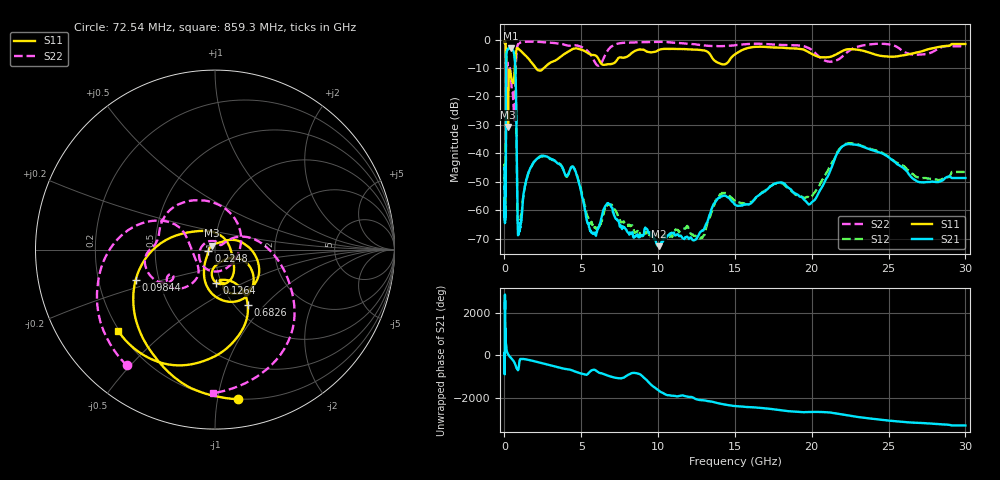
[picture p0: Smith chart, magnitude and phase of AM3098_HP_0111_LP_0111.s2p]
! Date/Time: Thu, Feb 28, 2019 8:38 AM
! Network Analyzer: Agilent Technologies E8364B Rev: A.07.50.67
! Sweep from 0.010 to 30.000 GHz, 1601 Points, Sweep Type: LOG
! Power Supply: 5.023 V, 0.001 A
# Hz S DB R 50
!freq MagS11 AngS11 MagS21 AngS21 MagS12 AngS12 MagS22 AngS22
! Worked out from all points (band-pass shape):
!   1601 points, 10 MHz to 30 GHz, reference 50 ohm
!   highest |S21| = -3.11 dB at 418 MHz (marker M1); lowest = -72.6 dB at 10.03 GHz (marker M2)
!   |S21| within 3 dB of the highest: 121.3 MHz to 660.5 MHz (539.2 MHz wide, 138 % of centre)
!   lowest |S11| = -30.7 dB at 231.6 MHz (marker M3), VSWR 1.06, Z = 48.1 + j2.15 ohm
!   |S11| at or under -10 dB: 102.2 MHz to 671.5 MHz (569.3 MHz wide, 147 % of centre); 2.04 GHz to 2.554 GHz (513.5 MHz wide, 22.4 % of centre)
!   |S22| runs from -28.3 to -0.6 dB; largest |S21 - S12| = 0.011
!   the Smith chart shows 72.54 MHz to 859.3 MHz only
!   S11 on the Smith chart (normalised r, x): 72.54 MHz: 0.20, -1.15; 98.44 MHz: 0.37, -0.16; 126.4 MHz: 0.95, -0.36; 224.8 MHz: 0.93, -0.01; 682.6 MHz: 1.14, -0.80; 859.3 MHz: 0.20, -0.35
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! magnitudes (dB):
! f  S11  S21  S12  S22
! 10 MHz  -0.3  -45.5  -44.7  -0.6
! 38.04 MHz  -0.4  -60.1  -61.2  -0.9
! 72.54 MHz  -1.5  -52.9  -52.1  -1.8
! 86.43 MHz  -2.8  -51.3  -51.7  -2.9
! 98.44 MHz  -6.5  -27.2  -27.2  -7.3
! 126.4 MHz  -14.7  -5.5  -5.4  -9.8
! 144.7 MHz  -20.0  -4.2  -4.1  -11.2
! 182.2 MHz  -10.5  -3.8  -3.8  -8.0
! 224.8 MHz  -28.6  -3.3  -3.3  -9.3
! 231.6 MHz  -30.7  -3.3  -3.2  -9.5
! 418 MHz  -12.6  -3.1  -3.1  -13.3
! 550.5 MHz  -15.2  -3.8  -3.7  -19.4
! 682.6 MHz  -9.0  -7.5  -7.5  -20.5
! 859.3 MHz  -3.0  -63.8  -63.6  -1.9
! 2.084 GHz  -10.3  -42.0  -42.0  -0.8
! 4.48 GHz  -3.3  -44.7  -44.8  -2.0
! 5.725 GHz  -5.4  -67.9  -65.2  -6.3
! 7.926 GHz  -6.1  -66.7  -65.3  -1.1
! 10.03 GHz  -3.7  -72.6  -68.9  -0.8
! 19.9 GHz  -4.7  -57.8  -55.7  -3.3
! 22.56 GHz  -3.4  -36.7  -36.4  -3.5
! 30 GHz  -1.6  -48.6  -46.5  -2.3
